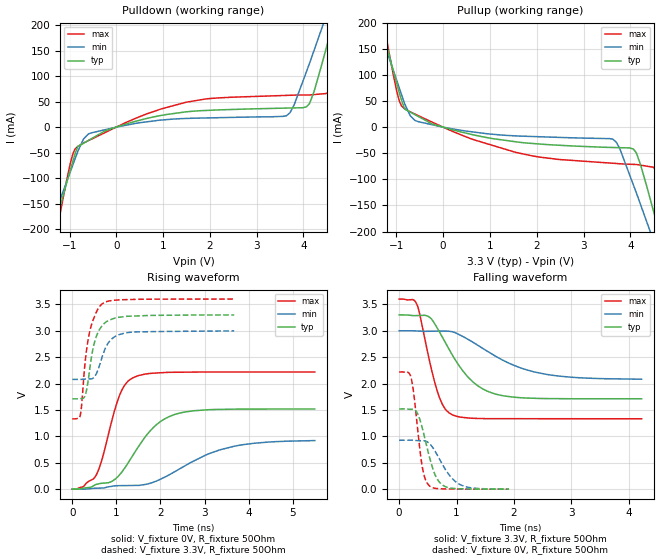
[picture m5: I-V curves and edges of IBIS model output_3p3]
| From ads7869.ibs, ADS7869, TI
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|   output_3p3 Model
[Model]   output_3p3
Model_type   Output
Polarity   Non-Inverting
Vmeas = 1.65
Vref = 1.65
Cref = 30pF
Rref = 50
|   typ   min   max
|   (nom PVT)   (fast PVT)   (slow PVT)
|C_comp from frequency sweep method (F=8MHz)
|C_comp   3.511e-12   3.452e-12   3.655e-12
|ON state : BUFFER OUTPUT TURNED HIGH
|C_comp   3.511e-12   3.452e-12   3.655e-12
|OFF state: BUFFER OUTPUT TURNED LOW
|C_comp   3.341e-12   3.119e-12   3.570e-12
|C_comp from LC tank measurement(L=1nH)
|Resonant Frequency(Hz)   2.990e+09   3.030e+09   2.950e+09
C_comp   2.836e-12   2.762e-12   2.914e-12
|ON state : BUFFER OUTPUT TURNED HIGH
|Resonant Frequency(Hz)   2.990e+09   3.030e+09   2.950e+09
|C_comp   2.836e-12   2.762e-12   2.914e-12
|OFF state: BUFFER OUTPUT TURNED LOW
|Resonant Frequency(Hz)   2.970e+09   3.050e+09   2.900e+09
|C_comp   2.875e-12   2.726e-12   3.015e-12
| Where nom  PVT is Nominal Process, 3.3V, 36C
|   Fast PVT is Strong Process,  3.6V, -40C
|   Slow PVT is Weak Process,   3V, 96C
[Voltage Range]   3.3   3   3.6
|Ambient Temperature   25   85   -40
|Junction Temperature
[Temperature Range]   36   96   -40
[Pullup Reference]   3.3   3   3.6
[Pulldown Reference]   0   0   0
[Power Clamp Reference]   3.3   3   3.6
[GND Clamp Reference]   0   0   0
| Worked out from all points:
|   slope of the pulldown table from 0 to 0.495 V, typ, clamps not added: 36.9 ohm
|   slope of the pullup table from 0 to 0.495 V, typ, clamps not added: 42.6 ohm
|   falling waveform, V_fixture 3.3V, R_fixture 50Ohm: 20-80 % time 588ps typ, 971ps min, 295ps max; typ from 3.3 V to 1.71 V
|   rising waveform, V_fixture 0V, R_fixture 50Ohm: 20-80 % time 797ps typ, 1.33ns min, 442ps max; typ from 0 V to 1.52 V
|   rising waveform, V_fixture 3.3V, R_fixture 50Ohm: 20-80 % time 235ps typ, 272ps min, 218ps max; typ from 1.71 V to 3.3 V
|   falling waveform, V_fixture 0V, R_fixture 50Ohm: 20-80 % time 225ps typ, 325ps min, 141ps max; typ from 1.52 V to 0.001 V
[Pulldown]
|   Voltage   I(typ)   I(min)   I(max)
-3.3V     -851.1mA   -668.4mA   -1.149A
-1.061V   -109.4mA   -107.3mA   -104.4mA
-884.4mV  -53.69mA   -63.06mA   -43.52mA
-537mV    -22.97mA   -11.38mA   -23.87mA
1.492V    30.05mA    17.07mA    48.91mA
3.639V    37.43mA    22.61mA    62.34mA
3.798V    37.76mA    43.2mA     62.82mA
4.122V    45.48mA    123.3mA    63.17mA
4.399V    125.5mA    196mA      65.32mA
4.559V    180mA      238mA      75mA
4.793V    259.9mA    299.4mA    171.7mA
6.6V      876.3mA    773.9mA    1.02A
[Pullup]
|   Voltage   I(typ)   I(min)   I(max)
-3.3V     875.9mA    695.4mA    1.16A
-1.082V   113.3mA    112.9mA    107.7mA
-888mV    51.52mA    61.84mA    40.27mA
-537mV    20.69mA    10.61mA    22.19mA
1.549V    -28.01mA   -16.75mA   -48.27mA
3.63V     -38.96mA   -23.29mA   -69.15mA
4.122V    -48.5mA    -124.2mA   -71.51mA
4.356V    -115mA     -182.7mA   -74.79mA
4.494V    -160.4mA   -217.3mA   -76.82mA
4.62V     -201.8mA   -248.8mA   -106.6mA
4.76V     -248mA     -283.9mA   -167.5mA
6.6V      -853.1mA   -744.2mA   -1.019A
[Ramp]
R_load = 50
|   typ   min   max
dV/dt_r   0.911118/7.97396e-10   0.551895/1.32546e-09   1.33129/4.42232e-10
dV/dt_f   0.953346/5.8819e-10   0.552387/9.7718e-10   1.36055/2.95269e-10
[Falling Waveform]
V_fixture = 3.3V
V_fixture_min = 3V
V_fixture_max = 3.6V
R_fixture = 50Ohm
|   Time   V(typ)   V(min)   V(max)
0s        3.3V       3V         3.6V
310.1ps   3.288V     2.996V     3.496V
527.4ps   3.257V     2.99V      2.438V
680.9ps   3.019V     2.993V     1.803V
802.9ps   2.78V      2.994V     1.519V
921.8ps   2.55V      2.983V     1.411V
1.306ns   2.011V     2.768V     1.342V
1.765ns   1.779V     2.467V     1.335V
2.684ns   1.715V     2.155V     1.335V
4.224ns   1.712V     2.083V     1.333V
[Rising Waveform]
V_fixture = 0V
V_fixture_min = 0V
V_fixture_max = 0V
R_fixture = 50Ohm
|   Time   V(typ)   V(min)   V(max)
0s        856pV      10.16nV    722.1pV
248.2ps   17.54mV    1.471mV    46.06mV
537.7ps   88.13mV    17.67mV    259.1mV
680.9ps   112mV      21.55mV    582.7mV
1.073ns   273.2mV    66.28mV    1.779V
1.377ns   643.7mV    70.06mV    2.11V
1.883ns   1.202V     145.9mV    2.199V
2.434ns   1.441V     383.8mV    2.214V
3.674ns   1.515V     813.1mV    2.218V
5.5ns     1.519V     919.8mV    2.219V
[Rising Waveform]
V_fixture = 3.3V
V_fixture_min = 3V
V_fixture_max = 3.6V
R_fixture = 50Ohm
|   Time   V(typ)   V(min)   V(max)
0s        1.711V     2.079V     1.332V
182.4ps   1.714V     2.079V     1.4V
290.4ps   1.769V     2.084V     2.394V
355.4ps   2.028V     2.088V     2.81V
428.5ps   2.464V     2.088V     3.092V
527.4ps   2.846V     2.157V     3.317V
680.9ps   3.099V     2.513V     3.511V
857.7ps   3.206V     2.814V     3.567V
1.185ns   3.268V     2.954V     3.589V
3.674ns   3.299V     2.997V     3.6V
[Falling Waveform]
V_fixture = 0V
V_fixture_min = 0V
V_fixture_max = 0V
R_fixture = 50Ohm
|   Time   V(typ)   V(min)   V(max)
0s        1.519V     926.2mV    2.219V
156.6ps   1.515V     928.3mV    2.212V
214ps     1.513V     928.1mV    2.081V
305.1ps   1.463V     921.5mV    1.313V
399.6ps   1.171V     918.3mV    444.9mV
509.6ps   685mV      881.8mV    83.12mV
650.1ps   217.8mV    674.2mV    13.88mV
813.9ps   44.36mV    359.9mV    5.766mV
1.126ns   6.996mV    57.98mV    1.15mV
1.914ns   1.227mV    3.139mV    943.2uV
